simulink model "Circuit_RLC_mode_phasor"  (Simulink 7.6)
settings: Solver=ode23t  StartTime=0.0  StopTime=0.02  RelTol=1e-3
InitFcn:
  | clc
  | close all
  | delete *.mat
StopFcn:
  | load Ampl_Phase_VC2.mat
  | plot(y(1,:),y(2,:),y(1,:),y(3,:))
  | grid
  | axis([0 0.02 -150 150])
  | title('Amplitude et phase - Vc2')
  | xlabel('temps')
undefined symbols (not defined in the file or in its folder): Angle, Magnitude
libraries: powerlib x11

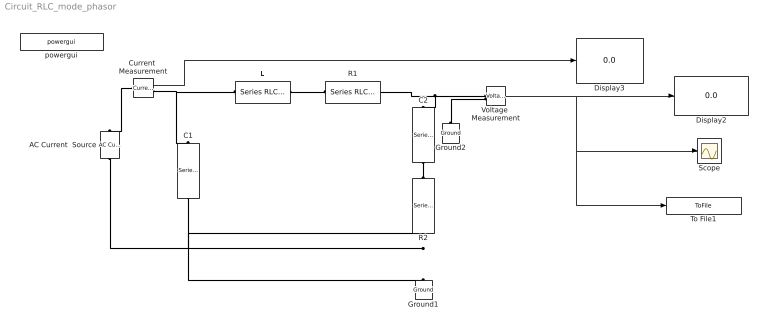
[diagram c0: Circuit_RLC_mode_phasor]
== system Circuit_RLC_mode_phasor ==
  AC Current  Source : powerlib/Electrical Sources/AC Current Source  DialogController=POWERSYS.PowerSysDialog  SystemSampleTime=-1  Amplitude=100  Phase=-30  Frequency=1000/(2*pi)  SampleTime=0  Measurements=None
  C1 : powerlib/Elements/Series RLC Branch  DialogController=POWERSYS.PowerSysDialog  PhysicalDomain=powersysdomain  SubClassName=unknown  LeftPortType=p1  RightPortType=p1  LConnTagsString=__new0  RConnTagsString=__new0  BranchType=C  Resistance=1  Inductance=1e-3  SetiL0=off  InitialCurrent=0  Capacitance=0.001  Setx0=off  InitialVoltage=0  Measurements=None
  C2 : powerlib/Elements/Series RLC Branch  DialogController=POWERSYS.PowerSysDialog  PhysicalDomain=powersysdomain  SubClassName=unknown  LeftPortType=p1  RightPortType=p1  LConnTagsString=__new0  RConnTagsString=__new0  BranchType=C  Resistance=1  Inductance=1e-3  SetiL0=off  InitialCurrent=0  Capacitance=0.001  Setx0=off  InitialVoltage=0  Measurements=None
  Current  Measurement : powerlib/Measurements/Current Measurement  DialogController=POWERSYS.PowerSysDialog  SystemSampleTime=-1  PhasorSimulation=on  OutputType=Magnitude-Angle  PSBequivalent=0
  Display2 : Display
  Display3 : Display
  Ground1 : powerlib/Elements/Ground  DialogController=POWERSYS.PowerSysDialog  PhysicalDomain=powersysdomain  SubClassName=unknown  LeftPortType=p1  RightPortType=p1  LConnTagsString=a
  Ground2 : powerlib/Elements/Ground  DialogController=POWERSYS.PowerSysDialog  PhysicalDomain=powersysdomain  SubClassName=unknown  LeftPortType=p1  RightPortType=p1  LConnTagsString=a
  L : powerlib/Elements/Series RLC Branch  DialogController=POWERSYS.PowerSysDialog  PhysicalDomain=powersysdomain  SubClassName=unknown  LeftPortType=p1  RightPortType=p1  LConnTagsString=__new0  RConnTagsString=__new0  BranchType=L  Resistance=4  Inductance=1e-3  SetiL0=off  InitialCurrent=0  Capacitance=0  Setx0=off  InitialVoltage=0  Measurements=None
  R1 : powerlib/Elements/Series RLC Branch  DialogController=POWERSYS.PowerSysDialog  PhysicalDomain=powersysdomain  SubClassName=unknown  LeftPortType=p1  RightPortType=p1  LConnTagsString=__new0  RConnTagsString=__new0  BranchType=R  Resistance=1  Inductance=10e-3  SetiL0=off  InitialCurrent=0  Capacitance=0  Setx0=off  InitialVoltage=0  Measurements=None
  R2 : powerlib/Elements/Series RLC Branch  DialogController=POWERSYS.PowerSysDialog  PhysicalDomain=powersysdomain  SubClassName=unknown  LeftPortType=p1  RightPortType=p1  LConnTagsString=__new0  RConnTagsString=__new0  BranchType=R  Resistance=1  Inductance=10e-3  SetiL0=off  InitialCurrent=0  Capacitance=0  Setx0=off  InitialVoltage=0  Measurements=None
  Scope : Scope
  To File1 : ToFile  Filename=Ampl_Phase_VC2  MatrixName=y
  Voltage  Measurement : powerlib/Measurements/Voltage Measurement  DialogController=POWERSYS.PowerSysDialog  SystemSampleTime=-1  PhasorSimulation=on  OutputType=Magnitude-Angle  PSBequivalent=0
  powergui : powerlib/powergui  Priority=1  SystemSampleTime=-1  SimulationMode=Phasor  SampleTime=50e-6  frequency=1000/(2*pi)  SPID=off  DisableSnubberDevices=off  DisableRonSwitches=off  DisableVfSwitches=off  SwTol=0  Interpol=off  frequencyindice=159.154943091895  echomessages=off  HookPort=off  DisplayEquations=off  FunctionMessages=off  EnableUseOfTLC=off  x0status=blocks  RestoreLinks=warning  ResistiveCurrentMeasurement=off  Frange=[0:2:500]  Ylog=off  Xlog=on  ShowGrid=on  save=off  variable=ZData  ZoomFFT=off  StartTime=0.0  cycles=1  DisplayStyle=1  fundamental=60  FreqAxis=off  MaxFrequency=1000  frequencyindicesteady=1  display=off  methode=off
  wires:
  Current  Measurement/1 -> Display3/1
  Voltage  Measurement/1 -> Display2/1, Scope/1, To File1/1
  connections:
  Current  Measurement/RConn1 -- C1/LConn1 -- L/LConn1
  Voltage  Measurement/LConn1 -- C2/LConn1 -- R1/RConn1
  Ground1/LConn1 -- R2/LConn1 -- C1/RConn1 -- AC Current  Source/LConn1
  Ground2/LConn1 -- Voltage  Measurement/LConn2
  Current  Measurement/LConn1 -- AC Current  Source/RConn1
  C2/RConn1 -- R2/RConn1
  R1/LConn1 -- L/RConn1
